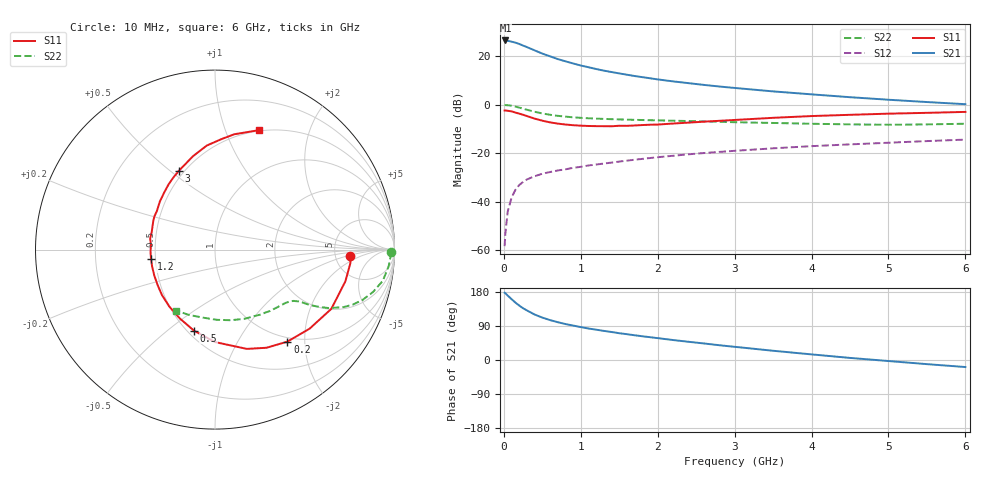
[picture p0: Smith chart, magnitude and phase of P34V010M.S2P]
! SIEMENS Small Signal Semiconductors
! BFP181
! Si NPN RF Bipolar Junction Transistor in SOT143
! VCE = 4 V  IC = 10 mA
! Common Emitter S-Parameters:  March  1996
# GHz  S  MA  R  50
!  f  S11  S21  S12  S22
! GHz  MAG  ANG  MAG  ANG  MAG  ANG  MAG  ANG
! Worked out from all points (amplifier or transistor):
!   36 points, 10 MHz to 6 GHz, reference 50 ohm
!   highest |S21| = 26.5 dB at 20 MHz (marker M1)
!   |S21| within 3 dB of that: start of sweep to 319.7 MHz
!   unconditionally stable (mu >= 1): 1.194 GHz to end of sweep
!   at 250 MHz: K = 0.33, MSG = 28.1 dB, |S12| = -31.9 dB
!   at 1.4 GHz: K = 1.07, MAG = 17.1 dB, |S12| = -23.9 dB
!   at 6 GHz: K = 1.00, MAG = 7.1 dB, |S12| = -14.4 dB
!   S11 on the Smith chart (normalised r, x): 10 MHz: 6.95, -1.24; 200 MHz: 0.93, -1.66; 500 MHz: 0.54, -0.62; 1.2 GHz: 0.47, -0.06; 3 GHz: 0.47, +0.54; 6 GHz: 0.49, +1.31
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0.01  0.7555 -2.9  21.03 177.6  0.0012 89.9  0.9812 -0.9
0.02  0.7584 -5.6  21.13 176.1  0.0022 81.2  0.9798 -2.0
0.05  0.7475 -13.7  20.8 170.0  0.0062 86.2  0.9722 -5.4
0.1  0.7274 -27.0  19.98 160.7  0.012 77.1  0.9512 -10.5
0.15  0.6869 -39.9  19.05 151.6  0.0174 69.7  0.9117 -15.0
0.2  0.6523 -51.8  17.9 143.7  0.0219 66.7  0.8691 -18.8
0.25  0.6177 -62.3  16.57 136.6  0.0254 62.7  0.8263 -21.8
0.3  0.581 -72.2  15.42 130.8  0.0286 59.4  0.7846 -24.1
0.4  0.5152 -90.0  13.19 120.0  0.0333 54.9  0.7129 -27.2
0.5  0.4666 -104.5  11.32 111.9  0.0375 51.9  0.6589 -28.9
0.6  0.4308 -117.1  9.956 105.4  0.0407 50.4  0.6187 -30.1
0.7  0.4066 -128.8  8.721 99.8  0.0438 49.6  0.5882 -30.8
0.9  0.3767 -147.5  7.085 90.9  0.0497 48.9  0.5478 -31.8
1.1  0.3628 -164.9  5.918 83.1  0.0556 48.9  0.5233 -33.1
1.2  0.3602 -171.4  5.44 80.0  0.0581 48.5  0.5153 -33.9
1.7  0.3715 159.6  3.898 65.3  0.073 48.0  0.486 -38.8
2.2  0.4077 138.9  3.021 52.7  0.0881 46.2  0.4659 -45.2
3  0.483 114.6  2.211 34.8  0.1114 41.4  0.4341 -57.8
3.5  0.5345 103.3  1.878 24.4  0.1255 37.8  0.4189 -67.0
4.5  0.6169 86.6  1.425 5.5  0.1514 30.1  0.3914 -88.5
5.5  0.6775 74.9  1.132 -10.9  0.1771 23.2  0.3913 -111.3
6  0.7084 69.9  1.022 -18.6  0.1898 19.0  0.4038 -122.8
